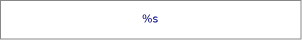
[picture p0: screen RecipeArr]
VISUALIZATION RecipeArr  // 302x40
VAR_INPUT
	ID:				INT;
END_VAR
    Rectangle (0,0 300x38), "%s", text variable: .strRecipeArr[ID], colour toggle: vbtRecipeArr[ID]
        OnMouseDown: execute { iSelectIndex:=ID; }
END_VISUALIZATION
